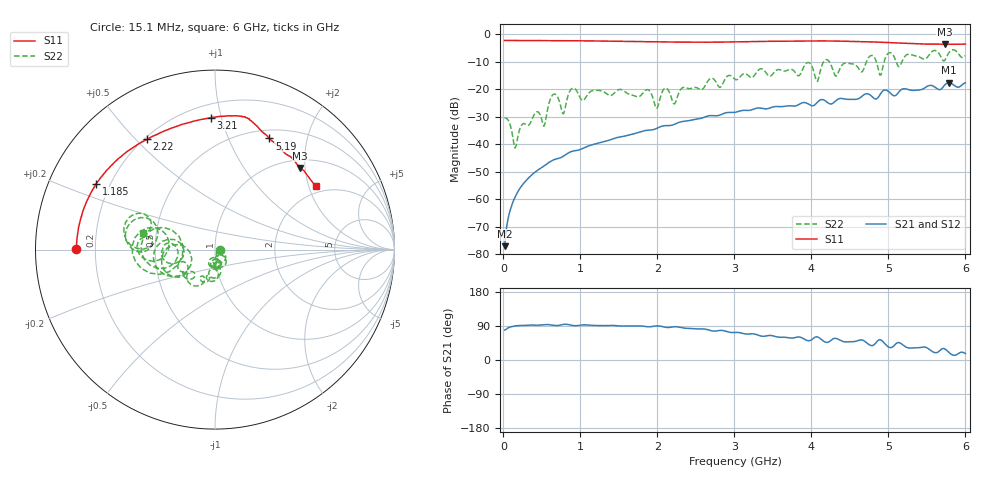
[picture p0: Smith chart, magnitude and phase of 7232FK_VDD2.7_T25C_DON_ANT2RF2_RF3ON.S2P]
!Agilent Technologies,E5071C,MY46417908,A.11.23
!Date: Fri Mar 03 11:29:54 2017
!Data & Calibration Information:
!Freq	S11:SOLT2(ON)	S21:SOLT2(ON)	S12:SOLT2(ON)	S22:SOLT2(ON)
!PortZ  Port1:50+j0  Port2:50+j0
!Above PortZ is port z conversion or system Z0 setting when saving the data.
!When reading, reference impedance value at option line is always used.
# Hz S dB R 50
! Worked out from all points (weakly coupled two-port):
!   400 points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, 15.1 MHz to 6 GHz, reference 50 ohm
!   highest |S21| = -17.64 dB at 5.79 GHz (marker M1); lowest = -77.1 dB at 15.1 MHz (marker M2)
!   lowest |S11| = -3.6 dB at 5.73 GHz (marker M3), VSWR 4.84, Z = 58.8 + j94.3 ohm
!   |S11| at or under -10 dB: nowhere
!   |S22| runs from -41.4 to -5.6 dB; largest |S21 - S12| = 0.0026
!   S11 on the Smith chart (normalised r, x): 15.1 MHz: 0.13, +0.00; 1.185 GHz: 0.15, +0.25; 2.22 GHz: 0.21, +0.54; 3.21 GHz: 0.29, +0.93; 5.19 GHz: 0.60, +1.42; 6 GHz: 1.78, +2.24
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1.509975e7  -2.24 179.6  -77.11 79.1  -77.13 78.0  -30.48 -8.6
1.500975e8  -2.25 176.5  -59.30 89.8  -59.32 90.0  -41.43 -42.9
2.550958e8  -2.26 174.3  -54.49 91.2  -54.47 91.3  -32.55 -34.7
5.250912e8  -2.29 167.9  -47.95 93.0  -47.96 93.1  -33.48 -52.2
6.450892e8  -2.30 164.9  -45.78 91.9  -45.78 91.8  -21.91 -47.0
7.80087e8  -2.33 161.6  -44.32 94.0  -44.34 94.1  -28.98 -60.1
8.850852e8  -2.34 159.0  -42.64 91.7  -42.65 91.8  -19.79 -56.5
1.020083e9  -2.38 155.5  -41.65 92.4  -41.68 92.3  -24.01 -79.4
1.18508e9  -2.43 151.2  -39.95 91.1  -39.95 91.1  -20.39 -77.7
2.010066e9  -2.75 128.2  -34.00 90.0  -34.00 90.0  -25.87 -76.6
2.100065e9  -2.78 125.5  -33.24 86.4  -33.24 86.4  -19.56 -88.4
2.220063e9  -2.84 121.6  -32.77 87.9  -32.77 87.9  -25.38 -83.6
3.01505e9  -2.75 96.8  -28.35 72.7  -28.34 72.8  -16.49 -106.3
3.210046e9  -2.66 91.6  -27.59 69.0  -27.57 69.0  -15.69 -116.5
4.005033e9  -2.43 78.4  -26.01 54.0  -25.99 53.7  -11.52 177.9
4.78502e9  -2.77 71.3  -22.60 37.9  -22.55 37.9  -7.68 177.1
4.890018e9  -2.91 69.5  -21.99 53.7  -21.97 53.2  -14.89 172.6
5.010016e9  -3.01 68.1  -20.98 33.5  -20.92 33.6  -6.74 -177.2
5.190014e9  -3.23 63.9  -19.84 39.4  -19.79 39.7  -9.12 -169.3
5.730004e9  -3.64 43.8  -18.49 29.6  -18.45 30.0  -9.56 172.1
5.790004e9  -3.58 41.8  -17.64 19.2  -17.57 19.9  -6.52 176.9
6e9  -3.55 32.0  -17.65 17.2  -17.61 18.1  -7.74 167.1
